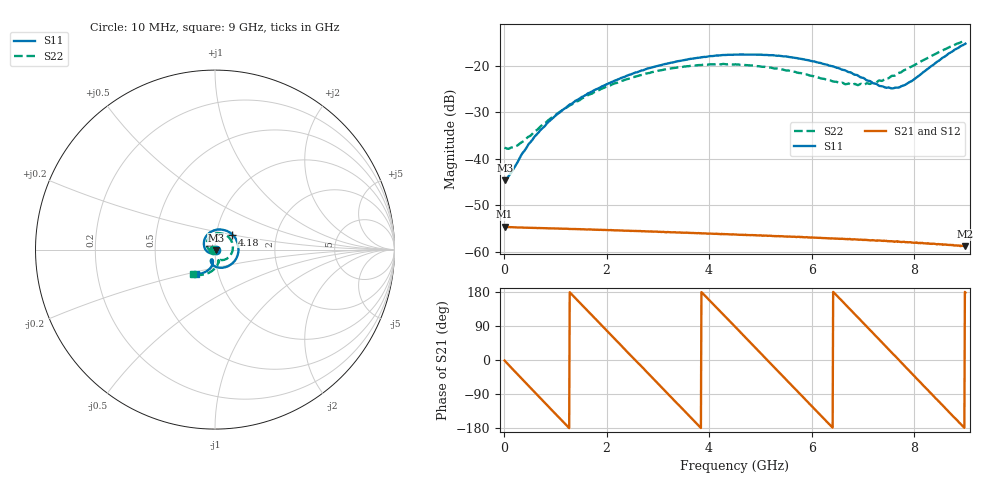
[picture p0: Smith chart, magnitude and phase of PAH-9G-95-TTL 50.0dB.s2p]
! MTS Systemtechnik GmbH
! S-Parameters
! Model: PAH-9G/95-TTL
! Attenuation Step: 50.0dB
#  HZ  S  DB  R  50.00
! Rohde & Schwarz Vector Network Analyzer
! Rohde-Schwarz,ZNB20-2Port,1334333062101652,3.45
! Created: UTC 1/26/2024, 7:22:13 AM
! freq[Hz]  db:S11  ang:S11  db:S21  ang:S21  db:S12  ang:S12  db:S22  ang:S22
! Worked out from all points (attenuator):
!   900 points, 10 MHz to 9 GHz, reference 50 ohm
!   highest |S21| = -54.65 dB at 10 MHz (marker M1); lowest = -58.8 dB at 9 GHz (marker M2)
!   lowest |S11| = -44.6 dB at 20 MHz (marker M3), VSWR 1.01, Z = 50.6 - j0.174 ohm
!   |S11| at or under -10 dB: start of sweep to end of sweep
!   |S22| runs from -37.9 to -14.6 dB; largest |S21 - S12| = 5.7e-05
!   S11 on the Smith chart (normalised r, x): 10 MHz: 1.01, -0.00; 4.18 GHz: 1.20, +0.20; 9 GHz: 0.78, -0.22
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1e7  -44.23 -22.8  -54.65 -1.4  -54.69 -1.3  -37.61 -170.3
2e7  -44.64 -17.1  -54.69 -3.0  -54.72 -3.1  -37.69 -174.7
7e7  -44.08 -23.3  -54.71 -10.2  -54.75 -10.3  -37.89 -176.5
2.5e8  -41.02 -61.5  -54.79 -35.9  -54.83 -36.0  -37.24 -169.1
4.7e8  -37.02 -89.3  -54.87 -67.2  -54.89 -67.1  -35.34 -164.5
7.1e8  -33.85 -111.3  -54.91 -100.9  -54.98 -100.9  -33.07 -167.0
1.02e9  -30.64 -135.1  -55.01 -144.7  -55.05 -144.6  -30.51 -176.1
1.51e9  -26.79 -166.5  -55.19 146.5  -55.23 146.8  -27.13 163.2
2.14e9  -23.35 156.0  -55.41 58.3  -55.44 58.5  -23.92 133.7
3.01e9  -20.04 106.8  -55.75 -63.0  -55.78 -63.4  -21.11 91.4
3.63e9  -18.59 71.8  -55.97 -150.0  -55.97 -149.5  -20.09 61.6
4.18e9  -17.86 40.8  -56.18 133.1  -56.22 133.5  -19.72 35.3
4.51e9  -17.67 22.1  -56.31 87.4  -56.35 87.6  -19.75 19.3
5.21e9  -17.79 -18.6  -56.57 -10.7  -56.64 -9.7  -20.46 -13.7
6.01e9  -19.08 -63.9  -56.96 -122.8  -56.98 -121.6  -22.24 -47.4
6.54e9  -20.62 -91.0  -57.22 163.1  -57.25 164.5  -23.78 -63.1
6.9e9  -22.13 -104.9  -57.41 112.8  -57.42 114.1  -24.22 -68.8
7.51e9  -24.74 -108.5  -57.78 27.2  -57.74 28.6  -22.67 -75.2
7.69e9  -24.74 -104.0  -57.83 2.1  -57.90 3.3  -21.63 -78.6
7.85e9  -23.98 -100.9  -57.95 -21.1  -57.98 -19.0  -20.83 -82.8
8.46e9  -19.12 -105.2  -58.38 -106.3  -58.41 -104.3  -17.24 -106.7
9e9  -15.31 -127.1  -58.82 177.8  -58.87 179.7  -14.62 -131.8
